| TEXAS INSTRUMENTS INCORPORATED
| Standard Linear and Logic Group
| IBIS Model of SN74LVCH16245A
| 16 Bit Bus Transceiver With 3 State Outputs
| This file contains package information for the following:
|  TSSOP 48-pin (DGG) package as [Component] LVCH16245A_DGG
|  SSOP 48-pin (DL) package as [Component] LVCH16245A_DL
|  TVSOP 48-pin (DGV) package as [Component] LVCH16245A_DGV
|  UFBGA 48-pin (GQL) package as [Component] LVCH16245A_GQL
|  UFBGA 48-pin (ZQL) package as [Component] LVCH16245A_ZQL
| This device can be powered at the following Vccs:
|  3.3 volt Vcc
|  2.5 volt Vcc
|  1.8 volt Vcc
| This file provides unique models under the [Model Selector] for each Vcc.
| For operation at a specific Vcc, select the appropriate model after each
| [Model Selector] keyword.
[IBIS Ver]   3.2
[Comment char]  |_char
[File Name]   sn74lvch16245a.ibs
[File Rev]   1.2 | d_die
[Date]   March 23, 2005
[Source]   Data created from TI-SPICE simulations at TI-SLL.
[Notes]   The following is an IBIS list for the LVCH16245A.
   Please contact sllibis@ti.com with questions and
   comments concerning SLL IBIS models.
   - FILE REV HISTORY
   - 1.1 Release IBIS file on 03/08/02
   - 1.2 GQL and ZQL packages added and file updated on 03/23/05
   - As there is no power clamp diode in the Input and I/O
   Models, we removed the Pwr Clamp table data from those Models.
   - Due to BUS-HOLD Circuit, there are non-monotonic
   warnings in I/O GND Clamp curve. Bus-Hold currents
   are not accurate in the I/O model.
   - Due to the fact that the Device is 5-V Input/Output
   tolarent, the output model has some Non-Monotonic Warnings.
   - C_comp values are taken at a different test condition than
   the data sheet.
   - There is one end point warnings in the file which could be
   avoided. Data was taken at higher load than 100 ohms
[Disclaimer] Property of Texas Instruments Incorporated.  Unauthorized
   reproduction and/or distribution is strictly prohibited.
   This product is protected under copyright law.
   Created  2001, (C) Copyright  2001, Texas Instruments
   Incorporated, All Rights Reserved
   UNLESS THERE IS A SIGNED, WRITTEN AGREEMENT TO THE
   CONTRARY, TEXAS INSTRUMENTS (TI) IS PROVIDING THE IBIS
   MODELS  AND WITHOUT ANY WARRANTY, EXPRESSED OR
   IMPLIED.  TI assumes no liability for:
   1) the accuracy of the IBIS models provided to your
   company;
   2) the proper functioning of these IBIS Models in your
   design or for any resulting applications; or
   3) infringement of patents, copyrights or intellectual
   property rights resulting from your use of these IBIS
   models.
   TI provides IBIS Models as a service to our customers.
   You and your company shall not distribute, sell or give
   these models to anyone else without prior written
   permission from TI.
   TI reserves the right to make changes to our products or
   to discontinue any semiconductor product or service
   without notice, and advises our customers to obtain the
   latest version of relevant information to verify, before
   placing orders, that the information being relied on is
   current.
   Please be aware that your receipt and use of the IBIS
   information provided shall serve as acceptance of these
   terms and conditions.  If you do not accept these terms,
   you should return or destroy the IBIS models and any
   other accompanying information immediately.
| Component LVCH16245A_DGG 48-pin TSSOP
[Component]   LVCH16245A_DGG
[Manufacturer]   Texas Instruments, Inc.
[Package]
|   typ   min   max
R_pkg   6.200e-02   5.000e-02   7.800e-02
L_pkg   3.527e-09   3.128e-09   4.255e-09
C_pkg   5.300e-13   4.170e-13   6.850e-13
[Pin]   signal_name   model_name   R_pin   L_pin   C_pin
1   1DIR   LVCH16245A_DIRIN   5.000e-02   4.250e-09   6.710e-13
2   1B1   LVCH16245A_IO   5.700e-02   3.956e-09   6.740e-13
3   1B2   LVCH16245A_IO   7.100e-02   3.922e-09   6.190e-13
4   GND   GND   7.800e-02   3.841e-09   6.180e-13
5   1B3   LVCH16245A_IO   5.600e-02   3.535e-09   5.550e-13
6   1B4   LVCH16245A_IO   5.800e-02   3.464e-09   5.030e-13
7   VCC   POWER   6.000e-02   3.362e-09   4.980e-13
8   1B5   LVCH16245A_IO   6.100e-02   3.293e-09   4.620e-13
9   1B6   LVCH16245A_IO   6.300e-02   3.240e-09   4.550e-13
10   GND   GND   6.300e-02   3.175e-09   4.420e-13
11   1B7   LVCH16245A_IO   6.400e-02   3.153e-09   4.290e-13
12   1B8   LVCH16245A_IO   6.500e-02   3.128e-09   4.180e-13
13   2B1   LVCH16245A_IO   6.500e-02   3.128e-09   4.180e-13
14   2B2   LVCH16245A_IO   6.400e-02   3.154e-09   4.290e-13
15   GND   GND   6.300e-02   3.174e-09   4.420e-13
16   2B3   LVCH16245A_IO   6.300e-02   3.241e-09   4.550e-13
17   2B4   LVCH16245A_IO   6.100e-02   3.293e-09   4.620e-13
18   VCC   POWER   6.000e-02   3.362e-09   4.970e-13
19   2B5   LVCH16245A_IO   5.800e-02   3.464e-09   5.030e-13
20   2B6   LVCH16245A_IO   5.600e-02   3.537e-09   5.600e-13
21   GND   GND   7.700e-02   3.839e-09   6.260e-13
22   2B7   LVCH16245A_IO   7.100e-02   3.917e-09   6.270e-13
23   2B8   LVCH16245A_IO   5.800e-02   3.955e-09   6.850e-13
24   2DIR   LVCH16245A_DIRIN   5.200e-02   4.255e-09   6.790e-13
25   2OE   LVCH16245A_OEIN   5.100e-02   4.254e-09   6.760e-13
26   2A8   LVCH16245A_IO   5.800e-02   3.957e-09   6.790e-13
27   2A7   LVCH16245A_IO   7.100e-02   3.920e-09   6.210e-13
28   GND   GND   7.800e-02   3.843e-09   6.220e-13
29   2A6   LVCH16245A_IO   5.600e-02   3.539e-09   5.600e-13
30   2A5   LVCH16245A_IO   5.800e-02   3.466e-09   5.030e-13
31   VCC   POWER   6.000e-02   3.363e-09   4.970e-13
32   2A4   LVCH16245A_IO   6.100e-02   3.294e-09   4.620e-13
33   2A3   LVCH16245A_IO   6.300e-02   3.241e-09   4.540e-13
34   GND   GND   6.300e-02   3.175e-09   4.410e-13
35   2A2   LVCH16245A_IO   6.400e-02   3.153e-09   4.290e-13
36   2A1   LVCH16245A_IO   6.500e-02   3.129e-09   4.170e-13
37   1A8   LVCH16245A_IO   6.500e-02   3.129e-09   4.170e-13
38   1A7   LVCH16245A_IO   6.400e-02   3.152e-09   4.290e-13
39   GND   GND   6.400e-02   3.176e-09   4.410e-13
40   1A6   LVCH16245A_IO   6.300e-02   3.241e-09   4.540e-13
41   1A5   LVCH16245A_IO   6.100e-02   3.293e-09   4.620e-13
42   VCC   POWER   6.000e-02   3.363e-09   4.970e-13
43   1A4   LVCH16245A_IO   5.800e-02   3.464e-09   5.030e-13
44   1A3   LVCH16245A_IO   5.600e-02   3.534e-09   5.610e-13
45   GND   GND   7.800e-02   3.841e-09   6.260e-13
46   1A2   LVCH16245A_IO   7.100e-02   3.920e-09   6.220e-13
47   1A1   LVCH16245A_IO   5.700e-02   3.955e-09   6.770e-13
48   1OE   LVCH16245A_OEIN   5.100e-02   4.252e-09   6.720e-13
| Component LVCH16245A_DL 48-pin SSOP
[Component]   LVCH16245A_DL
[Manufacturer]   Texas Instruments, Inc.
[Package]
|   typ   min   max
R_pkg   4.800e-02   3.800e-02   5.300e-02
L_pkg   6.046e-09   5.084e-09   7.968e-09
C_pkg   8.130e-13   5.690e-13   1.157e-12
[Pin]   signal_name   model_name   R_pin   L_pin   C_pin
1   1DIR   LVCH16245A_DIRIN   4.600e-02   7.968e-09   1.017e-12
2   1B1   LVCH16245A_IO   4.400e-02   7.299e-09   1.157e-12
3   1B2   LVCH16245A_IO   4.300e-02   6.765e-09   1.058e-12
4   GND   GND   4.100e-02   6.269e-09   9.330e-13
5   1B3   LVCH16245A_IO   3.800e-02   5.856e-09   8.290e-13
6   1B4   LVCH16245A_IO   4.600e-02   5.802e-09   7.900e-13
7   VCC   POWER   5.000e-02   5.656e-09   7.380e-13
8   1B5   LVCH16245A_IO   5.300e-02   5.500e-09   6.430e-13
9   1B6   LVCH16245A_IO   5.200e-02   5.304e-09   6.060e-13
10   GND   GND   5.300e-02   5.189e-09   5.830e-13
11   1B7   LVCH16245A_IO   5.100e-02   5.084e-09   5.690e-13
12   1B8   LVCH16245A_IO   5.300e-02   5.862e-09   8.330e-13
13   2B1   LVCH16245A_IO   5.300e-02   5.862e-09   8.330e-13
14   2B2   LVCH16245A_IO   5.100e-02   5.084e-09   5.690e-13
15   GND   GND   5.300e-02   5.189e-09   5.830e-13
16   2B3   LVCH16245A_IO   5.200e-02   5.304e-09   6.060e-13
17   2B4   LVCH16245A_IO   5.300e-02   5.500e-09   6.430e-13
18   VCC   POWER   5.000e-02   5.656e-09   7.380e-13
19   2B5   LVCH16245A_IO   4.600e-02   5.802e-09   7.900e-13
20   2B6   LVCH16245A_IO   3.800e-02   5.856e-09   8.290e-13
21   GND   GND   4.100e-02   6.269e-09   9.330e-13
22   2B7   LVCH16245A_IO   4.300e-02   6.765e-09   1.058e-12
23   2B8   LVCH16245A_IO   4.400e-02   7.299e-09   1.157e-12
24   2DIR   LVCH16245A_DIRIN   4.600e-02   7.968e-09   1.017e-12
25   2OE   LVCH16245A_OEIN   4.600e-02   7.968e-09   1.017e-12
26   2A8   LVCH16245A_IO   4.400e-02   7.299e-09   1.157e-12
27   2A7   LVCH16245A_IO   4.300e-02   6.765e-09   1.058e-12
28   GND   GND   4.100e-02   6.269e-09   9.330e-13
29   2A6   LVCH16245A_IO   3.800e-02   5.856e-09   8.290e-13
30   2A5   LVCH16245A_IO   4.600e-02   5.802e-09   7.900e-13
31   VCC   POWER   5.000e-02   5.656e-09   7.380e-13
32   2A4   LVCH16245A_IO   5.300e-02   5.500e-09   6.430e-13
33   2A3   LVCH16245A_IO   5.200e-02   5.304e-09   6.060e-13
34   GND   GND   5.300e-02   5.189e-09   5.830e-13
35   2A2   LVCH16245A_IO   5.100e-02   5.084e-09   5.690e-13
36   2A1   LVCH16245A_IO   5.300e-02   5.862e-09   8.330e-13
37   1A8   LVCH16245A_IO   5.300e-02   5.862e-09   8.330e-13
38   1A7   LVCH16245A_IO   5.100e-02   5.084e-09   5.690e-13
39   GND   GND   5.300e-02   5.189e-09   5.830e-13
40   1A6   LVCH16245A_IO   5.200e-02   5.304e-09   6.060e-13
41   1A5   LVCH16245A_IO   5.300e-02   5.500e-09   6.430e-13
42   VCC   POWER   5.000e-02   5.656e-09   7.380e-13
43   1A4   LVCH16245A_IO   4.600e-02   5.802e-09   7.900e-13
44   1A3   LVCH16245A_IO   3.800e-02   5.856e-09   8.290e-13
45   GND   GND   4.100e-02   6.269e-09   9.330e-13
46   1A2   LVCH16245A_IO   4.300e-02   6.765e-09   1.058e-12
47   1A1   LVCH16245A_IO   4.400e-02   7.299e-09   1.157e-12
48   1OE   LVCH16245A_OEIN   4.600e-02   7.967e-09   1.017e-12
| Component LVCH16245A_DGV 48-pin TVSOP
[Component]   LVCH16245A_DGV
[Manufacturer]   Texas   Instruments,   Inc.
[Package]
|   typ   min   max
R_pkg   0.07   0.049   0.085
L_pkg   3.01E-09   2.74E-09   3.41E-09
C_pkg   3.71E-13   2.94E-13   5.11E-13
[Pin]   signal_name   model_name   R_pin   L_pin   C_pin
1   1DIR   LVCH16245A_DIRIN   0.049   3.39E-09   4.97E-13
2   1B1   LVCH16245A_IO   0.06   3.25E-09   5.02E-13
3   1B2   LVCH16245A_IO   0.077   3.31E-09   4.51E-13
4   GND   GND   0.085   3.3E-09   4.04E-13
5   1B3   LVCH16245A_IO   0.083   3.14E-09   3.6E-13
6   1B4   LVCH16245A_IO   0.077   3.02E-09   3.63E-13
7   VCC   POWER   0.065   2.88E-09   3.49E-13
8   1B5   LVCH16245A_IO   0.066   2.83E-09   3.14E-13
9   1B6   LVCH16245A_IO   0.067   2.8E-09   3.14E-13
10   GND   GND   0.069   2.75E-09   3.08E-13
11   1B7   LVCH16245A_IO   0.07   2.75E-09   3.01E-13
12   1B8   LVCH16245A_IO   0.071   2.75E-09   2.94E-13
13   2B1   LVCH16245A_IO   0.07   2.74E-09   2.94E-13
14   2B2   LVCH16245A_IO   0.07   2.75E-09   3.01E-13
15   GND   GND   0.069   2.75E-09   3.08E-13
16   2B3   LVCH16245A_IO   0.067   2.8E-09   3.14E-13
17   2B4   LVCH16245A_IO   0.066   2.83E-09   3.14E-13
18   VCC   POWER   0.065   2.88E-09   3.5E-13
19   2B5   LVCH16245A_IO   0.075   3.01E-09   3.63E-13
20   2B6   LVCH16245A_IO   0.08   3.13E-09   3.58E-13
21   GND   GND   0.084   3.3E-09   4.03E-13
22   2B7   LVCH16245A_IO   0.078   3.31E-09   4.52E-13
23   2B8   LVCH16245A_IO   0.062   3.26E-09   5.01E-13
24   2DIR   LVCH16245A_DIRIN   0.052   3.4E-09   4.96E-13
25   2OE   LVCH16245A_OEIN   0.053   3.4E-09   5.05E-13
26   2A8   LVCH16245A_IO   0.062   3.25E-09   5.11E-13
27   2A7   LVCH16245A_IO   0.077   3.31E-09   4.53E-13
28   GND   GND   0.082   3.29E-09   4.03E-13
29   2A6   LVCH16245A_IO   0.078   3.12E-09   3.59E-13
30   2A5   LVCH16245A_IO   0.074   3.01E-09   3.63E-13
31   VCC   POWER   0.065   2.88E-09   3.49E-13
32   2A4   LVCH16245A_IO   0.067   2.83E-09   3.14E-13
33   2A3   LVCH16245A_IO   0.067   2.8E-09   3.14E-13
34   GND   GND   0.069   2.75E-09   3.07E-13
35   2A2   LVCH16245A_IO   0.07   2.75E-09   3.01E-13
36   2A1   LVCH16245A_IO   0.07   2.74E-09   2.94E-13
37   1A8   LVCH16245A_IO   0.07   2.74E-09   2.94E-13
38   1A7   LVCH16245A_IO   0.07   2.75E-09   3.01E-13
39   GND   GND   0.069   2.75E-09   3.07E-13
40   1A6   LVCH16245A_IO   0.068   2.8E-09   3.14E-13
41   1A5   LVCH16245A_IO   0.067   2.83E-09   3.14E-13
42   VCC   POWER   0.064   2.88E-09   3.49E-13
43   1A4   LVCH16245A_IO   0.072   3E-09   3.62E-13
44   1A3   LVCH16245A_IO   0.078   3.12E-09   3.59E-13
45   GND   GND   0.084   3.3E-09   4.03E-13
46   1A2   LVCH16245A_IO   0.077   3.31E-09   4.51E-13
47   1A1   LVCH16245A_IO   0.062   3.26E-09   4.99E-13
48   1OE   LVCH16245A_OEIN   0.053   3.41E-09   4.94E-13
| Component LVCH16245A_GQL 48-pin UFBGA
[Component]   LVCH16245A_GQL
[Manufacturer]   Texas Instruments, Inc.
[Package]
|   typ   min   max
R_pkg   7.900e-02   4.500e-02   9.400e-02
L_pkg   2.264e-09   1.398e-09   2.722e-09
C_pkg   3.060e-13   1.170e-13   4.040e-13
[Pin]   signal_name   model_name   R_pin   L_pin   C_pin
A1   1DIR   LVCH16245A_DIRIN   5.100e-02   1.531e-09   2.100e-13
B2   1B1   LVCH16245A_IO   7.300e-02   2.572e-09   3.120e-13
B1   1B2   LVCH16245A_IO   7.100e-02   1.835e-09   2.320e-13
B3   GND   GND   9.400e-02   2.717e-09   3.830e-13
C2   1B3   LVCH16245A_IO   8.900e-02   2.534e-09   3.500e-13
C1   1B4   LVCH16245A_IO   7.100e-02   1.831e-09   2.310e-13
C3   VCC   POWER   9.400e-02   2.722e-09   3.920e-13
D2   1B5   LVCH16245A_IO   9.000e-02   2.551e-09   3.520e-13
D1   1B6   LVCH16245A_IO   7.200e-02   1.846e-09   2.440e-13
D3   GND   GND   9.400e-02   2.719e-09   4.030e-13
E2   1B7   LVCH16245A_IO   8.900e-02   2.541e-09   3.510e-13
E1   1B8   LVCH16245A_IO   7.200e-02   1.850e-09   2.270e-13
F1   2B1   LVCH16245A_IO   7.200e-02   1.850e-09   2.270e-13
F2   2B2   LVCH16245A_IO   8.900e-02   2.541e-09   3.510e-13
G3   GND   GND   9.400e-02   2.718e-09   4.040e-13
G1   2B3   LVCH16245A_IO   7.200e-02   1.847e-09   2.440e-13
G2   2B4   LVCH16245A_IO   9.000e-02   2.551e-09   3.520e-13
H3   VCC   POWER   9.400e-02   2.721e-09   3.920e-13
H1   2B5   LVCH16245A_IO   7.000e-02   1.830e-09   2.310e-13
H2   2B6   LVCH16245A_IO   8.800e-02   2.524e-09   3.500e-13
J3   GND   GND   9.300e-02   2.709e-09   3.820e-13
J1   2B7   LVCH16245A_IO   7.100e-02   1.851e-09   2.330e-13
J2   2B8   LVCH16245A_IO   5.600e-02   2.605e-09   3.900e-13
K1   2DIR   LVCH16245A_DIRIN   4.500e-02   1.398e-09   1.170e-13
K6   2OE   LVCH16245A_OEIN   4.500e-02   1.512e-09   1.930e-13
J5   2A8   LVCH16245A_IO   5.500e-02   2.492e-09   3.130e-13
J6   2A7   LVCH16245A_IO   7.000e-02   1.821e-09   2.300e-13
J4   GND   GND   9.300e-02   2.703e-09   3.820e-13
H5   2A6   LVCH16245A_IO   8.900e-02   2.529e-09   3.500e-13
H6   2A5   LVCH16245A_IO   7.100e-02   1.826e-09   2.300e-13
H4   VCC   POWER   9.400e-02   2.722e-09   3.910e-13
G5   2A4   LVCH16245A_IO   9.000e-02   2.551e-09   3.520e-13
G6   2A3   LVCH16245A_IO   7.200e-02   1.846e-09   2.440e-13
G4   GND   GND   9.400e-02   2.719e-09   4.040e-13
F5   2A2   LVCH16245A_IO   8.800e-02   2.510e-09   3.490e-13
F6   2A1   LVCH16245A_IO   7.200e-02   1.850e-09   2.270e-13
E6   1A8   LVCH16245A_IO   7.100e-02   1.850e-09   2.270e-13
E5   1A7   LVCH16245A_IO   8.900e-02   2.529e-09   3.500e-13
D4   GND   GND   9.400e-02   2.719e-09   4.030e-13
D6   1A6   LVCH16245A_IO   7.200e-02   1.847e-09   2.430e-13
D5   1A5   LVCH16245A_IO   8.900e-02   2.550e-09   3.520e-13
C4   VCC   POWER   9.400e-02   2.722e-09   3.910e-13
C6   1A4   LVCH16245A_IO   7.100e-02   1.827e-09   2.300e-13
C5   1A3   LVCH16245A_IO   8.900e-02   2.539e-09   3.500e-13
B4   GND   GND   9.300e-02   2.705e-09   3.820e-13
B6   1A2   LVCH16245A_IO   7.100e-02   1.831e-09   2.270e-13
B5   1A1   LVCH16245A_IO   7.300e-02   2.685e-09   3.800e-13
A6   1OE   LVCH16245A_OEIN   5.100e-02   1.417e-09   1.330e-13
| Component LVCH16245A_ZQL 48-pin UFBGA
[Component]   LVCH16245A_ZQL
[Manufacturer]   Texas Instruments, Inc.
[Package]
|   typ   min   max
R_pkg   7.900e-02   4.500e-02   9.400e-02
L_pkg   2.264e-09   1.398e-09   2.722e-09
C_pkg   3.060e-13   1.170e-13   4.040e-13
[Pin]   signal_name   model_name   R_pin   L_pin   C_pin
A1   1DIR   LVCH16245A_DIRIN   5.100e-02   1.531e-09   2.100e-13
B2   1B1   LVCH16245A_IO   7.300e-02   2.572e-09   3.120e-13
B1   1B2   LVCH16245A_IO   7.100e-02   1.835e-09   2.320e-13
B3   GND   GND   9.400e-02   2.717e-09   3.830e-13
C2   1B3   LVCH16245A_IO   8.900e-02   2.534e-09   3.500e-13
C1   1B4   LVCH16245A_IO   7.100e-02   1.831e-09   2.310e-13
C3   VCC   POWER   9.400e-02   2.722e-09   3.920e-13
D2   1B5   LVCH16245A_IO   9.000e-02   2.551e-09   3.520e-13
D1   1B6   LVCH16245A_IO   7.200e-02   1.846e-09   2.440e-13
D3   GND   GND   9.400e-02   2.719e-09   4.030e-13
E2   1B7   LVCH16245A_IO   8.900e-02   2.541e-09   3.510e-13
E1   1B8   LVCH16245A_IO   7.200e-02   1.850e-09   2.270e-13
F1   2B1   LVCH16245A_IO   7.200e-02   1.850e-09   2.270e-13
F2   2B2   LVCH16245A_IO   8.900e-02   2.541e-09   3.510e-13
G3   GND   GND   9.400e-02   2.718e-09   4.040e-13
G1   2B3   LVCH16245A_IO   7.200e-02   1.847e-09   2.440e-13
G2   2B4   LVCH16245A_IO   9.000e-02   2.551e-09   3.520e-13
H3   VCC   POWER   9.400e-02   2.721e-09   3.920e-13
H1   2B5   LVCH16245A_IO   7.000e-02   1.830e-09   2.310e-13
H2   2B6   LVCH16245A_IO   8.800e-02   2.524e-09   3.500e-13
J3   GND   GND   9.300e-02   2.709e-09   3.820e-13
J1   2B7   LVCH16245A_IO   7.100e-02   1.851e-09   2.330e-13
J2   2B8   LVCH16245A_IO   5.600e-02   2.605e-09   3.900e-13
K1   2DIR   LVCH16245A_DIRIN   4.500e-02   1.398e-09   1.170e-13
K6   2OE   LVCH16245A_OEIN   4.500e-02   1.512e-09   1.930e-13
J5   2A8   LVCH16245A_IO   5.500e-02   2.492e-09   3.130e-13
J6   2A7   LVCH16245A_IO   7.000e-02   1.821e-09   2.300e-13
J4   GND   GND   9.300e-02   2.703e-09   3.820e-13
H5   2A6   LVCH16245A_IO   8.900e-02   2.529e-09   3.500e-13
H6   2A5   LVCH16245A_IO   7.100e-02   1.826e-09   2.300e-13
H4   VCC   POWER   9.400e-02   2.722e-09   3.910e-13
G5   2A4   LVCH16245A_IO   9.000e-02   2.551e-09   3.520e-13
G6   2A3   LVCH16245A_IO   7.200e-02   1.846e-09   2.440e-13
G4   GND   GND   9.400e-02   2.719e-09   4.040e-13
F5   2A2   LVCH16245A_IO   8.800e-02   2.510e-09   3.490e-13
F6   2A1   LVCH16245A_IO   7.200e-02   1.850e-09   2.270e-13
E6   1A8   LVCH16245A_IO   7.100e-02   1.850e-09   2.270e-13
E5   1A7   LVCH16245A_IO   8.900e-02   2.529e-09   3.500e-13
D4   GND   GND   9.400e-02   2.719e-09   4.030e-13
D6   1A6   LVCH16245A_IO   7.200e-02   1.847e-09   2.430e-13
D5   1A5   LVCH16245A_IO   8.900e-02   2.550e-09   3.520e-13
C4   VCC   POWER   9.400e-02   2.722e-09   3.910e-13
C6   1A4   LVCH16245A_IO   7.100e-02   1.827e-09   2.300e-13
C5   1A3   LVCH16245A_IO   8.900e-02   2.539e-09   3.500e-13
B4   GND   GND   9.300e-02   2.705e-09   3.820e-13
B6   1A2   LVCH16245A_IO   7.100e-02   1.831e-09   2.270e-13
B5   1A1   LVCH16245A_IO   7.300e-02   2.685e-09   3.800e-13
A6   1OE   LVCH16245A_OEIN   5.100e-02   1.417e-09   1.330e-13
| Model LVCH16245A_DIRIN
[Model Selector]   LVCH16245A_DIRIN
LVCH16245A_DIRIN_33   3.3 volt Vcc
LVCH16245A_DIRIN_25   2.5 volt Vcc
LVCH16245A_DIRIN_18   1.8 volt Vcc
| Model LVCH16245A_OEIN
[Model Selector]   LVCH16245A_OEIN
LVCH16245A_OEIN_33   3.3 volt Vcc
LVCH16245A_OEIN_25   2.5 volt Vcc
LVCH16245A_OEIN_18   1.8 volt Vcc
| Model LVCH16245A_IO
[Model Selector]   LVCH16245A_IO
LVCH16245A_IO_33   3.3 volt Vcc
LVCH16245A_IO_25   2.5 volt Vcc
LVCH16245A_IO_18   1.8 volt Vcc
| Models and submodels in the file (9): LVCH16245A_DIRIN_33 (Input), LVCH16245A_DIRIN_25 (Input), LVCH16245A_DIRIN_18 (Input), LVCH16245A_OEIN_33 (Input), LVCH16245A_OEIN_25 (Input), LVCH16245A_OEIN_18 (Input), LVCH16245A_IO_33 (3-state), LVCH16245A_IO_25 (3-state), LVCH16245A_IO_18 (3-state)
